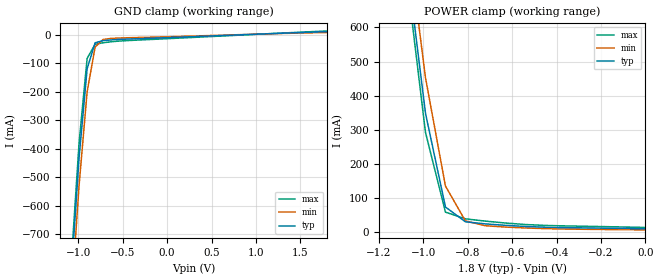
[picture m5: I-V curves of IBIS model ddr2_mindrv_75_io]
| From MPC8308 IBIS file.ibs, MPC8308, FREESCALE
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[Model]   ddr2_mindrv_75_io   |
Model_type   Input
Vinl = 0.87
Vinh = 0.93
| variable   typ   min   max
C_comp   1.17p   1.10p   1.23p
[Model Spec]
| subparameter   typ   min   max
S_overshoot_high  3.300   3.135   3.465
S_overshoot_low   -200.00m  -100.00m  -300.00m
D_overshoot_high  4.000   4.000   4.000
D_overshoot_low   -1.000   -1.000   -1.000
D_overshoot_time  1.000n   1.000n   1.000n
| variable   typ   min   max
[Temperature Range]   55.0   110.0   0.0
| variable   typ   min   max
[Pullup Reference]   1.800V   1.710V   1.890V
| variable   typ   min   max
[Pulldown Reference]   0.000V   0.000V   0.000V
| variable   typ   min   max
[POWER_Clamp_Reference]   1.800V   1.710V   1.890V
| variable   typ   min   max
[GND_Clamp_Reference]   0.000V   0.000V   0.000V
[GND_clamp]
|Voltage   I(typ)   I(min)   I(max)
-1.89V    -5.308A    -5.326A    -5.317A
-1.08V    -849.1mA   -937mA     -806.6mA
-990mV    -430mA     -527.3mA   -378.3mA
-900mV    -120mA     -201.2mA   -83.73mA
-810mV    -28.8mA    -43.87mA   -33.84mA
-720mV    -21.4mA    -17.15mA   -28.85mA
-630mV    -18.74mA   -13.53mA   -25.26mA
1.8V      10.14mA    7.342mA    12.67mA
[POWER_clamp]
|Voltage   I(typ)   I(min)   I(max)
-1.71V    4.954A     4.965A     4.97A
-1.08V    823.2mA    916.3mA    779mA
-990mV    349mA      453.2mA    292.9mA
-900mV    73.83mA    135.1mA    58.79mA
-810mV    30.41mA    32.91mA    39.11mA
-720mV    24.29mA    18.89mA    32.43mA
-450mV    14.55mA    10.43mA    19.75mA
-2.22fV   10.14mA    6.762mA    13.91mA
